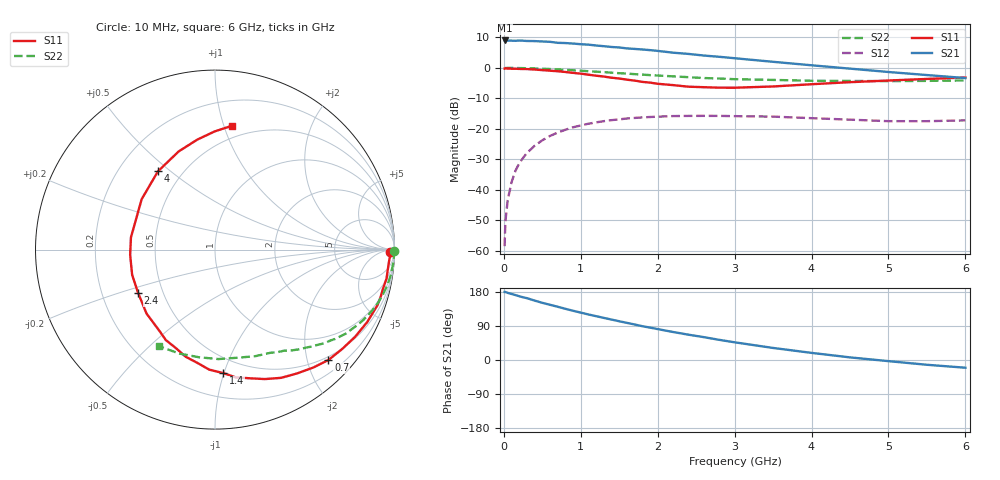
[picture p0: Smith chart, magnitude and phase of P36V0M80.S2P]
! SIEMENS Small Signal Semiconductors
! BFP181
! Si NPN RF Bipolar Junction Transistor in SOT143
! VCE = 6 V  IC = 0.8 mA
! Common Emitter S-Parameters:  March  1996
# GHz  S  MA  R  50
!  f  S11  S21  S12  S22
! GHz  MAG  ANG  MAG  ANG  MAG  ANG  MAG  ANG
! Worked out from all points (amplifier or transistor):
!   36 points, 10 MHz to 6 GHz, reference 50 ohm
!   highest |S21| = 9.0 dB at 10 MHz (marker M1)
!   |S21| within 3 dB of that: start of sweep to 1.82 GHz
!   unconditionally stable (mu >= 1): 3.46 GHz to end of sweep
!   at 250 MHz: K = 0.08, MSG = 19.2 dB, |S12| = -29.5 dB
!   at 1.4 GHz: K = 0.46, MSG = 12.0 dB, |S12| = -17.1 dB
!   at 6 GHz: K = 1.31, MAG = 3.6 dB, |S12| = -17.2 dB
!   S11 on the Smith chart (normalised r, x): 10 MHz: 59, -30; 700 MHz: 0.43, -2.40; 1.4 GHz: 0.38, -1.00; 2.4 GHz: 0.36, -0.23; 4 GHz: 0.37, +0.45; 6 GHz: 0.40, +1.06
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0.01  0.9735 -0.8  2.813 179.6  0.0012 83.5  0.9989 -0.3
0.02  0.9804 -1.4  2.801 179.5  0.003 91.0  0.9937 -0.5
0.05  0.9733 -3.0  2.803 177.2  0.0068 90.9  0.9972 -1.6
0.1  0.9692 -6.7  2.791 174.3  0.0134 85.5  0.9973 -3.0
0.15  0.9692 -9.6  2.776 171.4  0.0205 83.2  0.9951 -4.5
0.25  0.9597 -16.0  2.786 165.4  0.0335 79.6  0.9902 -7.7
0.3  0.9564 -19.0  2.758 163.2  0.0403 76.8  0.9873 -9.1
0.4  0.9391 -25.5  2.747 156.8  0.053 73.1  0.9795 -12.0
0.6  0.899 -38.1  2.672 145.7  0.0767 64.1  0.9567 -17.8
0.7  0.882 -44.2  2.572 140.5  0.087 60.2  0.9432 -20.5
0.9  0.8279 -56.4  2.501 129.9  0.1064 52.4  0.9141 -25.5
1.1  0.7732 -68.9  2.399 120.1  0.1217 45.6  0.8814 -30.2
1.4  0.6899 -86.1  2.199 106.7  0.1392 36.0  0.8344 -36.6
1.8  0.5896 -111.9  2.001 89.2  0.1544 26.2  0.7754 -43.4
2.2  0.5219 -137.0  1.774 73.9  0.1623 17.2  0.7265 -49.9
2.4  0.4916 -150.7  1.693 66.8  0.1634 13.3  0.7039 -53.0
3  0.4732 171.8  1.439 46.7  0.162 3.9  0.6528 -61.7
3.5  0.4958 145.5  1.257 31.8  0.159 -1.7  0.6348 -69.3
4  0.5396 126.1  1.103 18.8  0.15 -5.2  0.6154 -78.2
4.5  0.5832 110.3  0.972 6.9  0.1418 -7.6  0.6102 -88.2
5.5  0.6587 90.1  0.763 -12.6  0.1339 -4.2  0.6123 -109.0
6  0.6952 82.4  0.681 -20.4  0.1379 -2.2  0.6223 -119.9
